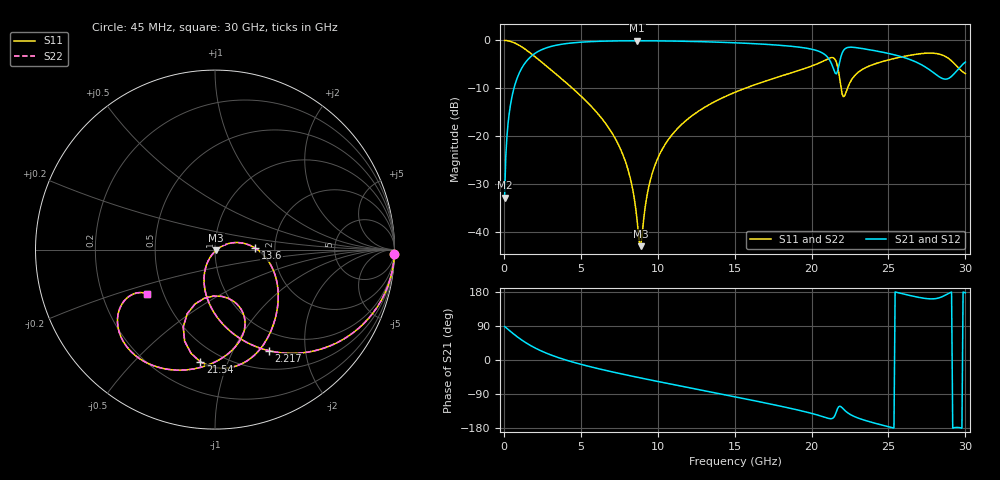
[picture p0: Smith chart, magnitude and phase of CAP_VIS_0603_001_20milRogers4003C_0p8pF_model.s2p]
! S-parameter model data by Modelithics Inc.  support@modelithics.com  813-866-6335  Tampa FL USA
! S-Parameter data specifications:
! Substrate: 20-mil Rogers 4003C, substrate thickness, H=0.508mm, Dielectric constant, Er=3.75
! PCB Mounting Pad Footprint: Pad width, PadW=0.90mm , Pad length, PadL=1.00mm , Pad gap, PadG (edge-to-edge)=1.00mm , Reference planes=3.0mm apart
! Created Wed Nov 18 13:17:04 2015
# hz S ma R 50
! 2 Port Network Data from SP1.SP block
! freq  magS11  angS11  magS21  angS21  magS12  angS12  magS22  angS22
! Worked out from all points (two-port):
!   401 points, 45 MHz to 30 GHz, reference 50 ohm
!   highest |S21| = -0.07 dB at 8.657 GHz (marker M1); lowest = -32.8 dB at 45 MHz (marker M2)
!   |S21| within 3 dB of the highest: 1.863 GHz to 20.91 GHz (19.05 GHz wide, 167 % of centre); 21.94 GHz to 25.47 GHz (3.532 GHz wide, 14.9 % of centre)
!   lowest |S11| = -42.9 dB at 8.882 GHz (marker M3), VSWR 1.01, Z = 50.5 - j0.479 ohm
!   |S11| at or under -10 dB: 4.468 GHz to 15.65 GHz (11.18 GHz wide, 111 % of centre); 21.92 GHz to 22.33 GHz (412.3 MHz wide, 1.86 % of centre)
!   |S22| runs from -42.9 to 0.0 dB; largest |S21 - S12| = 0
!   S11 on the Smith chart (normalised r, x): 45 MHz: 1, -74; 2.217 GHz: 0.73, -1.40; 13.6 GHz: 1.58, +0.02; 21.54 GHz: 0.39, -0.80; 30 GHz: 0.41, -0.25
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4.5e7  0.9997 -1.6  0.02297 88.4  0.02297 88.4  0.9997 -1.6
3.4455e8  0.9848 -11.8  0.1735 78.2  0.1735 78.2  0.9848 -11.8
6.441e8  0.9493 -21.7  0.3137 68.2  0.3137 68.2  0.9493 -21.7
2.216738e9  0.6389 -61.9  0.7665 27.9  0.7665 27.9  0.6389 -61.9
5.062462e9  0.2584 -100.9  0.9606 -12.0  0.9606 -12.0  0.2584 -100.9
7.608638e9  0.07204 -121.2  0.9903 -36.4  0.9903 -36.4  0.07204 -121.2
8.282625e9  0.03299 -120.3  0.9919 -42.3  0.9919 -42.3  0.03299 -120.3
8.657062e9  0.01341 -103.9  0.9922 -45.4  0.9922 -45.4  0.01341 -103.9
8.881725e9  0.00718 -41.3  0.9921 -47.3  0.9921 -47.3  0.00718 -41.3
9.480825e9  0.0331 24.7  0.9912 -52.3  0.9912 -52.3  0.0331 24.7
1.007992e10  0.06299 25.6  0.9894 -57.3  0.9894 -57.3  0.06299 25.6
1.359964e10  0.2257 1.9  0.9632 -85.7  0.9632 -85.7  0.2257 1.9
1.50225e10  0.2884 -9.3  0.9453 -97.1  0.9453 -97.1  0.2884 -9.3
2.003996e10  0.5435 -54.4  0.8081 -141.3  0.8081 -141.3  0.5435 -54.4
2.10135e10  0.6375 -71.8  0.677 -153.1  0.677 -153.1  0.6375 -71.8
2.153771e10  0.6311 -97.4  0.4555 -144.6  0.4555 -144.6  0.6311 -97.4
2.213681e10  0.2629 -82.1  0.8081 -132.1  0.8081 -132.1  0.2629 -82.1
2.296058e10  0.4555 -68.5  0.839 -152.2  0.839 -152.2  0.4555 -68.5
2.505742e10  0.6304 -90.8  0.7287 -176.7  0.7287 -176.7  0.6304 -90.8
2.707939e10  0.7277 -115.7  0.5656 164.4  0.5656 164.4  0.7277 -115.7
2.850225e10  0.7037 -139.4  0.4015 167.3  0.4015 167.3  0.7037 -139.4
3e10  0.4513 -146.8  0.5957 177.2  0.5957 177.2  0.4513 -146.8
